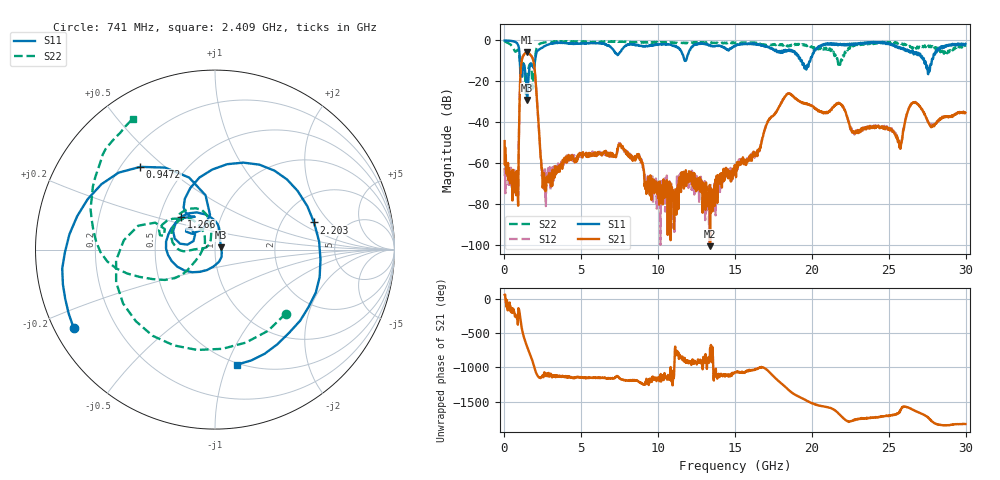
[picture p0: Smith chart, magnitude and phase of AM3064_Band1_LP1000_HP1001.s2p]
# Hz S DB R 50.0
!freq dBS11 angS11 dBS21 angS21 dBS12 angS12 dBS22 angS22
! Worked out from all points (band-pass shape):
!   1600 points, 10 MHz to 29.98 GHz, reference 50 ohm
!   highest |S21| = -5.82 dB at 1.453 GHz (marker M1); lowest = -100.5 dB at 13.37 GHz (marker M2)
!   |S21| within 3 dB of the highest: 1.155 GHz to 1.832 GHz (677.5 MHz wide, 45.4 % of centre)
!   lowest |S11| = -29.1 dB at 1.472 GHz (marker M3), VSWR 1.07, Z = 53.4 + j1.35 ohm
!   |S11| at or under -10 dB: 1.002 GHz to 1.99 GHz (988.6 MHz wide, 66.1 % of centre); 19.34 GHz to 19.89 GHz (545.5 MHz wide, 2.78 % of centre); 27.3 GHz to 27.8 GHz (495.7 MHz wide, 1.8 % of centre)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
!   |S22| runs from -27.2 to -0.3 dB; largest |S21 - S12| = 0.0061
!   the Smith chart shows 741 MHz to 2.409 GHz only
!   S11 on the Smith chart (normalised r, x): 741 MHz: 0.06, -0.26; 947.2 MHz: 0.28, +0.42; 1.266 GHz: 0.64, +0.25; 2.203 GHz: 3.01, +1.35; 2.409 GHz: 0.49, -1.09
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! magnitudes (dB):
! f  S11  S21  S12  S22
! 10 MHz  -0.1  -49.2  -62.4  -0.3
! 741 MHz  -0.9  -64.3  -74.9  -5.5
! 947.2 MHz  -4.1  -43.8  -43.6  -5.8
! 1.116 GHz  -15.3  -10.2  -10.2  -10.7
! 1.266 GHz  -11.6  -7.0  -7.0  -11.9
! 1.453 GHz  -25.9  -5.8  -5.8  -21.1
! 1.472 GHz  -29.1  -5.8  -5.8  -19.1
! 1.884 GHz  -13.3  -10.1  -10.2  -18.2
! 2.203 GHz  -4.9  -39.0  -39.0  -2.3
! 2.409 GHz  -3.7  -62.3  -62.1  -1.3
! 5.015 GHz  -1.4  -55.3  -56.2  -0.8
! 7.564 GHz  -5.4  -50.8  -51.0  -0.6
! 10 GHz  -2.0  -73.6  -73.1  -0.9
! 13.37 GHz  -2.4  -100.5  -69.4  -1.0
! 15 GHz  -2.8  -63.0  -62.6  -1.5
! 18.36 GHz  -5.4  -26.4  -26.4  -2.7
! 19.99 GHz  -8.2  -32.1  -32.2  -3.1
! 25 GHz  -1.3  -43.1  -42.7  -1.0
! 25.75 GHz  -3.5  -53.0  -51.6  -1.6
! 26.63 GHz  -6.9  -30.5  -30.3  -3.1
! 27.58 GHz  -14.6  -40.1  -40.0  -2.5
! 29.98 GHz  -1.7  -35.3  -35.2  -3.1
